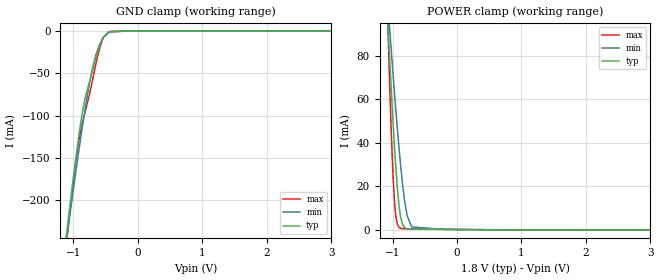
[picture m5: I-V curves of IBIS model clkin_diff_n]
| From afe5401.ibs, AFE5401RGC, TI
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[Model]   clkin_diff_n
Model_type   Input
Vinl = 0.45
Vinh = 1.35
|   (nom PVT)   (fast PVT)   (slow PVT)
C_comp   2.855e-12   2.445e-12   3.305e-12
[Model spec]
|subparameter
Vinl   0.45   0.425   0.475
Vinh   1.35   1.275   1.425
| Where nom  PVT is Nominal Process, 1.8V, 27C
|   Fast PVT is Strong Process,  1.9V, -40C
|   Slow PVT is Weak Process,   1.7V, 125C
[Voltage Range]   1.8   1.7   1.9
|Junction Temperature
[Temperature Range]   27   125   -40
[Power Clamp Reference]   1.8   1.7   1.9
[GND Clamp Reference]   0   0   0
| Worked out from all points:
|   GND clamp passes 1 mA (typ) near -0.45 V on its own axis
|   POWER clamp passes 1 mA (typ) near -0.81 V on its own axis
[GND Clamp]
|   Voltage   I(typ)   I(min)   I(max)
-1.8V     -724.2mA   -669.6mA   -781.4mA
-1.125V   -252.7mA   -258.5mA   -264.6mA
-1.029V   -190.8mA   -203.3mA   -197.2mA
-967.8mV  -153.9mA   -169.7mA   -158.4mA
-920.3mV  -126.9mA   -144.2mA   -132.6mA
-870.1mV  -101.2mA   -118.2mA   -112.2mA
-820.8mV  -80.83mA   -93.78mA   -96.63mA
-749.3mV  -59.98mA   -61.73mA   -74.84mA
-647.4mV  -30.73mA   -27.75mA   -37.94mA
-544.1mV  -8.321mA   -8.727mA   -9.354mA
-449.1mV  -1.074mA   -1.663mA   -947.9uA
3.6V      0A         0A         0A
[POWER Clamp]
|   Voltage   I(typ)   I(min)   I(max)
-1.8V     580.1mA    428.2mA    963.3mA
-1.074V   95.96mA    104.6mA    95.48mA
-1.042V   76.95mA    91.32mA    64.26mA
-1.008V   57.85mA    77.65mA    35.69mA
-986.8mV  46.81mA    69.47mA    21.75mA
-948.6mV  28.6mA     54.99mA    6.294mA
-895.6mV  10.15mA    36.37mA    1.089mA
-873mV    5.6mA      29.16mA    732.3uA
-813.6mV  1.105mA    13.45mA    542uA
-774.9mV  571.1uA    6.691mA    521.7uA
-703.5mV  392.7uA    1.422mA    498.8uA
3.6V      0A         0A         0A
